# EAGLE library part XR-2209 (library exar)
Precision OSCILLATOR
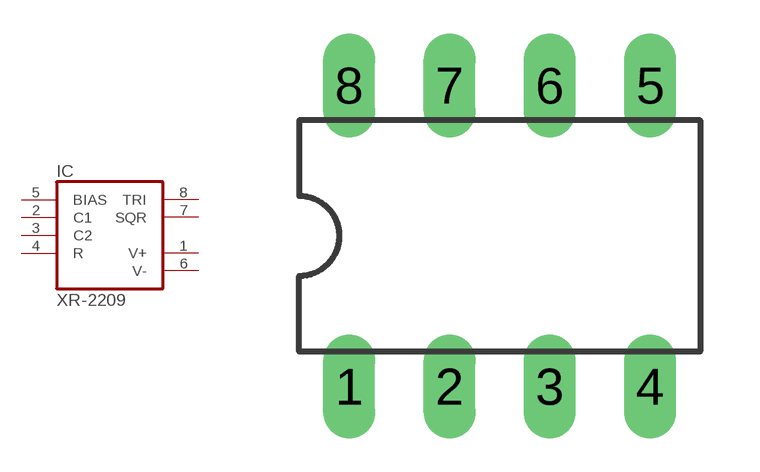
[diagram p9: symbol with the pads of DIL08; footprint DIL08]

Designator prefix IC

## XR-2209 (OC_FARNELL: unknown; OC_NEWARK: unknown)  [DIL08]
1  V+  pwr
2  C1  in
3  C2  in
4  R  in
5  BIAS  in
6  V-  pwr
7  SQR  out
8  TRI  out

## Footprint DIL08 (pad centres in mm)
Dual In Line Package
drill 0.813 long: 1 -3.81,-3.81; 2 -1.27,-3.81; 3 1.27,-3.81; 4 3.81,-3.81; 5 3.81,3.81; 6 1.27,3.81; 7 -1.27,3.81; 8 -3.81,3.81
